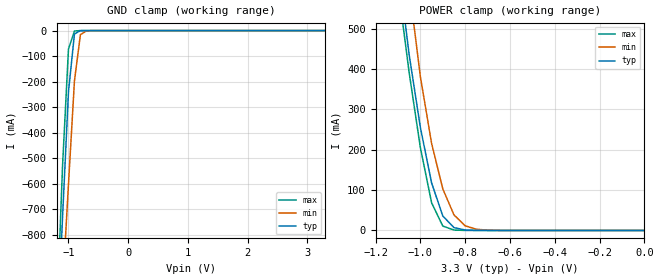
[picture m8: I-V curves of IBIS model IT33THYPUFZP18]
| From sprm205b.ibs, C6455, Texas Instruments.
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|   Model IT33THYPUFZP18
[Model]   IT33THYPUFZP18
Model_type   Input
Polarity   Non-Inverting
Vinl =   0.8000V
Vinh =   2.0000V
C_comp   0.5060pF   0.4600pF   0.5490pF
[Temperature Range]   25.0000   0.1250k   -40.0000
[Pullup Reference]   3.3000V   3.0000V   3.6000V
[Pulldown Reference]   0.000V   0.000V   0.000V
[POWER Clamp Reference]   3.3000V   3.0000V   3.6000V
[GND Clamp Reference]   0.000V   0.000V   0.000V
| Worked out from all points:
|   GND clamp passes 1 mA (typ) near -0.80 V on its own axis
|   POWER clamp passes 1 mA (typ) near -0.79 V on its own axis
[GND_clamp]
| voltage   I(typ)   I(min)   I(max)
-3.3V     -15.87A    -14.33A    -17.08A
-1.2V     -1.259A    -1.449A    -1.156A
-1.1V     -733.9mA   -1.017A    -533.5mA
-1V       -239.8mA   -601.8mA   -72.16mA
-900mV    -13.08mA   -197.2mA   -1.593mA
-800mV    -383.1uA   -15.95mA   -19.24uA
-700mV    -10.22uA   -1.076mA   -3.04uA
3.3V      95.96nA    1.337uA    329.8nA
[POWER_clamp]
| voltage   I(typ)   I(min)   I(max)
-3.3V     13.82A     12.46A     14.94A
-1.1V     659.5mA    849.4mA    605.1mA
-1.05V    434.5mA    602.9mA    390.3mA
-1V       254.9mA    380.7mA    204.9mA
-950mV    117.9mA    215.8mA    68.71mA
-900mV    35.9mA     103mA      10.9mA
-850mV    7.058mA    38.52mA    1.116mA
-800mV    1.156mA    11.51mA    138.8uA
-750mV    198.8uA    3.088mA    44.68uA
-700mV    48.89uA    806.8uA    30.59uA
0V        95.96nA    70.01nA    353.9nA
